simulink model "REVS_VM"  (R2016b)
settings: Solver=ode3  StartTime=REVS.sim_start_time_secs  StopTime=Inf  FixedStep=REVS.sim_step_time_secs  MaxStep=REVS.sim_step_time_secs  EnableMultiTasking=on
StopFcn:
  | postproc_datalog;
  | postproc_audit;
  | postproc_result;
model workspace (MATLAB code in the model file):
  other statements: REVS_setup_variants
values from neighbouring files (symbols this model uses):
  accessory = class_accessory_data    [class_test_data.m]
  battery = class_battery_data    [class_accessory_data.m]    (also in class_REVS_electric.m = class_REVS_battery)
  brake = struct(	'max_torque_Nm',[], 						'proportion_norm',1.0, 						'inertia_kgm2',0.0)    [class_REVS_drive_axle.m]
  engine = class_engine_data    [class_test_data.m]
  final_drive = struct(	'gear_ratio',[], 								'efficiency_norm',[], 								'inertia_kgm2',[] )    [class_REVS_drive_axle.m]
  gear = class_REVS_gearbox    [class_REVS_AT_transmission.m]
  tire = struct(	'radius_m',[], 						'rolling_resistance_coefficient',0, 						'vehicle_weight_norm',1.0,  						'wheel_slip_torque_Nm',[],  						'inertia_kgm2',0.0)    [class_REVS_drive_axle.m]
  torque_converter = class_REVS_torque_converter    [class_REVS_AT_transmission.m]
  transmission = class_transmission_data    [class_test_data.m]
  vehicle = class_vehicle_data    [class_test_data.m]
undefined symbols (not defined in the file or in its folder): alternator, ambient, controls, convert, DelayTimeSecs, drive_cycle, driver, electric, gear_strategy, InitialCondition, InitialValue, LoadSource, LookupStructure, MultiplyPosInputs, Normalize, NumPhases, REVS, SpeedSource, starter, tableshift, UpperSaturationLimit, Value, VerboseLevel, VerboseSignal
libraries: simulink x153
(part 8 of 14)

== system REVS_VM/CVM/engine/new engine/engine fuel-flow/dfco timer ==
  bool : Inport
  Constant : Constant  Value=Normalize
  Data Type Conversion2 : DataTypeConversion  OutDataTypeStr=double
  Integrator1 : Integrator  ExternalReset=falling  LimitOutput=on  UpperSaturationLimit=UpperSaturationLimit  LowerSaturationLimit=0
  Switch : Switch  Criteria=u2 > Threshold
  normalize : Gain  Gain=1/UpperSaturationLimit
  out : Outport
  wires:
  Switch/1 -> out/1
  normalize/1 -> Switch/1
  Integrator1/1 -> Switch/3, normalize/1
  Constant/1 -> Switch/2
  bool/1 -> Data Type Conversion2/1
  Data Type Conversion2/1 -> Integrator1/1, Integrator1/2

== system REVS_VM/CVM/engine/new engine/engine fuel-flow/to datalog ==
  Var : Inport
  Constant : Constant  Value=VerboseSignal
  Constant1 : Constant  Value=VerboseLevel
  Relational Operator : RelationalOperator  OutDataTypeStr=boolean  ZeroCross=off
  Subsystem : Subsystem
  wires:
  Constant1/1 -> Relational Operator/2
  Constant/1 -> Relational Operator/1
  Relational Operator/1 -> Subsystem/Enable
  Var/1 -> Subsystem/1(In1)

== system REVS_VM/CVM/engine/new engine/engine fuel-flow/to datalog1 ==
  Var : Inport
  Constant : Constant  Value=VerboseSignal
  Constant1 : Constant  Value=VerboseLevel
  Relational Operator : RelationalOperator  OutDataTypeStr=boolean  ZeroCross=off
  Subsystem : Subsystem
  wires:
  Constant1/1 -> Relational Operator/2
  Constant/1 -> Relational Operator/1
  Relational Operator/1 -> Subsystem/Enable
  Var/1 -> Subsystem/1(In1)

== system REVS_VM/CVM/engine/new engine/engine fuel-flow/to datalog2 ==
  Var : Inport
  Constant : Constant  Value=VerboseSignal
  Constant1 : Constant  Value=VerboseLevel
  Relational Operator : RelationalOperator  OutDataTypeStr=boolean  ZeroCross=off
  Subsystem : Subsystem
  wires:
  Constant1/1 -> Relational Operator/2
  Constant/1 -> Relational Operator/1
  Relational Operator/1 -> Subsystem/Enable
  Var/1 -> Subsystem/1(In1)

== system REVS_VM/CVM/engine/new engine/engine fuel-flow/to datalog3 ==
  Var : Inport
  Constant : Constant  Value=VerboseSignal
  Constant1 : Constant  Value=VerboseLevel
  Relational Operator : RelationalOperator  OutDataTypeStr=boolean  ZeroCross=off
  Subsystem : Subsystem
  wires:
  Constant1/1 -> Relational Operator/2
  Constant/1 -> Relational Operator/1
  Relational Operator/1 -> Subsystem/Enable
  Var/1 -> Subsystem/1(In1)

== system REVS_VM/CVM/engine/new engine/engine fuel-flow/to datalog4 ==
  Var : Inport
  Constant : Constant  Value=VerboseSignal
  Constant1 : Constant  Value=VerboseLevel
  Relational Operator : RelationalOperator  OutDataTypeStr=boolean  ZeroCross=off
  Subsystem : Subsystem
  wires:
  Constant1/1 -> Relational Operator/2
  Constant/1 -> Relational Operator/1
  Relational Operator/1 -> Subsystem/Enable
  Var/1 -> Subsystem/1(In1)

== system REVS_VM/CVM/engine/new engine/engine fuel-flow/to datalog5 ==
  Var : Inport
  Constant : Constant  Value=VerboseSignal
  Constant1 : Constant  Value=VerboseLevel
  Relational Operator : RelationalOperator  OutDataTypeStr=boolean  ZeroCross=off
  Subsystem : Subsystem
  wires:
  Constant1/1 -> Relational Operator/2
  Constant/1 -> Relational Operator/1
  Relational Operator/1 -> Subsystem/Enable
  Var/1 -> Subsystem/1(In1)

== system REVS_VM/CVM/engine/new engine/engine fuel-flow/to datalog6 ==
  Var : Inport
  Constant : Constant  Value=VerboseSignal
  Constant1 : Constant  Value=VerboseLevel
  Relational Operator : RelationalOperator  OutDataTypeStr=boolean  ZeroCross=off
  Subsystem : Subsystem
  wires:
  Constant1/1 -> Relational Operator/2
  Constant/1 -> Relational Operator/1
  Relational Operator/1 -> Subsystem/Enable
  Var/1 -> Subsystem/1(In1)

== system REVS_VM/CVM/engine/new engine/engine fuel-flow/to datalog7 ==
  Var : Inport
  Constant : Constant  Value=VerboseSignal
  Constant1 : Constant  Value=VerboseLevel
  Relational Operator : RelationalOperator  OutDataTypeStr=boolean  ZeroCross=off
  Subsystem : Subsystem
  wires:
  Constant1/1 -> Relational Operator/2
  Constant/1 -> Relational Operator/1
  Relational Operator/1 -> Subsystem/Enable
  Var/1 -> Subsystem/1(In1)

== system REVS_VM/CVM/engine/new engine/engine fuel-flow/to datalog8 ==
  Var : Inport
  Constant : Constant  Value=VerboseSignal
  Constant1 : Constant  Value=VerboseLevel
  Relational Operator : RelationalOperator  OutDataTypeStr=boolean  ZeroCross=off
  Subsystem : Subsystem
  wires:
  Constant1/1 -> Relational Operator/2
  Constant/1 -> Relational Operator/1
  Relational Operator/1 -> Subsystem/Enable
  Var/1 -> Subsystem/1(In1)

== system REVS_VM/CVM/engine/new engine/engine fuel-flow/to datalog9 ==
  Var : Inport
  Constant : Constant  Value=VerboseSignal
  Constant1 : Constant  Value=VerboseLevel
  Relational Operator : RelationalOperator  OutDataTypeStr=boolean  ZeroCross=off
  Subsystem : Subsystem
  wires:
  Constant1/1 -> Relational Operator/2
  Constant/1 -> Relational Operator/1
  Relational Operator/1 -> Subsystem/Enable
  Var/1 -> Subsystem/1(In1)

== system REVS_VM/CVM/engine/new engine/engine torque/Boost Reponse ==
  target_trq_Nm : Inport
  max_trq_Nm : Inport  Port=2
  nat_asp_trq_Nm : Inport  Port=3
  min_trq_Nm : Inport  Port=4
  Constant : Constant  Value=engine.boost_time_constant_secs
  Constant1 : Constant  Value=engine.boost_falling_time_constant_secs
  Dynamic Limit Integrator : Subsystem
  MinMax3 : MinMax  Function=max  Inputs=2  ZeroCross=off
  MinMax4 : MinMax  Inputs=2  ZeroCross=off
  Product : Product  Inputs=*/
  Sum : Sum  Inputs=|+-
  Sum1 : Sum  Inputs=|+-
  Switch : Switch  Criteria=u2 > Threshold
  trq_limit_Nm : Outport
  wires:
  min_trq_Nm/1 -> Sum1/2
  nat_asp_trq_Nm/1 -> Sum1/1
  Constant1/1 -> Switch/3
  Constant/1 -> Switch/1
  Switch/1 -> Product/2
  target_trq_Nm/1 -> MinMax3/1
  max_trq_Nm/1 -> Dynamic Limit Integrator/1(upper), MinMax4/1
  Sum1/1 -> MinMax3/2, Dynamic Limit Integrator/4(Xo), Dynamic Limit Integrator/5(lower)
  Product/1 -> Dynamic Limit Integrator/2(In)
  MinMax4/1 -> Sum/1
  Sum/1 -> Switch/2, Product/1
  MinMax3/1 -> MinMax4/2
  Dynamic Limit Integrator/1(Out) -> trq_limit_Nm/1, Sum/2

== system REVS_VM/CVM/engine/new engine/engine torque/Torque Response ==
  target_pow_W : Inport
  Constant : Constant  Value=1/engine.power_time_constant_secs
  Integrator : Integrator
  Product : Product
  Sum : Sum  Inputs=|+-
  act_pow_W : Outport
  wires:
  Product/1 -> Integrator/1
  Constant/1 -> Product/1
  Integrator/1 -> Sum/2, act_pow_W/1
  Sum/1 -> Product/2
  target_pow_W/1 -> Sum/1

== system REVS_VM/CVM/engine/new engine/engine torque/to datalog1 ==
  Var : Inport
  Constant : Constant  Value=VerboseSignal
  Constant1 : Constant  Value=VerboseLevel
  Relational Operator : RelationalOperator  OutDataTypeStr=boolean  ZeroCross=off
  Subsystem : Subsystem
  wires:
  Constant1/1 -> Relational Operator/2
  Constant/1 -> Relational Operator/1
  Relational Operator/1 -> Subsystem/Enable
  Var/1 -> Subsystem/1(In1)

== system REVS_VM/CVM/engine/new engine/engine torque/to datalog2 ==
  Var : Inport
  Constant : Constant  Value=VerboseSignal
  Constant1 : Constant  Value=VerboseLevel
  Relational Operator : RelationalOperator  OutDataTypeStr=boolean  ZeroCross=off
  Subsystem : Subsystem
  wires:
  Constant1/1 -> Relational Operator/2
  Constant/1 -> Relational Operator/1
  Relational Operator/1 -> Subsystem/Enable
  Var/1 -> Subsystem/1(In1)

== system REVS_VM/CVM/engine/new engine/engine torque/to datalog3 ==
  Var : Inport
  Constant : Constant  Value=VerboseSignal
  Constant1 : Constant  Value=VerboseLevel
  Relational Operator : RelationalOperator  OutDataTypeStr=boolean  ZeroCross=off
  Subsystem : Subsystem
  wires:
  Constant1/1 -> Relational Operator/2
  Constant/1 -> Relational Operator/1
  Relational Operator/1 -> Subsystem/Enable
  Var/1 -> Subsystem/1(In1)

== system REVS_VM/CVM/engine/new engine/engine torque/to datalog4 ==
  Var : Inport
  Constant : Constant  Value=VerboseSignal
  Constant1 : Constant  Value=VerboseLevel
  Relational Operator : RelationalOperator  OutDataTypeStr=boolean  ZeroCross=off
  Subsystem : Subsystem
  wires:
  Constant1/1 -> Relational Operator/2
  Constant/1 -> Relational Operator/1
  Relational Operator/1 -> Subsystem/Enable
  Var/1 -> Subsystem/1(In1)

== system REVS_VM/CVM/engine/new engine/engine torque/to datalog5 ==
  Var : Inport
  Constant : Constant  Value=VerboseSignal
  Constant1 : Constant  Value=VerboseLevel
  Relational Operator : RelationalOperator  OutDataTypeStr=boolean  ZeroCross=off
  Subsystem : Subsystem
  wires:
  Constant1/1 -> Relational Operator/2
  Constant/1 -> Relational Operator/1
  Relational Operator/1 -> Subsystem/Enable
  Var/1 -> Subsystem/1(In1)

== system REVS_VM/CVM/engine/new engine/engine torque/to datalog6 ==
  Var : Inport
  Constant : Constant  Value=VerboseSignal
  Constant1 : Constant  Value=VerboseLevel
  Relational Operator : RelationalOperator  OutDataTypeStr=boolean  ZeroCross=off
  Subsystem : Subsystem
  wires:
  Constant1/1 -> Relational Operator/2
  Constant/1 -> Relational Operator/1
  Relational Operator/1 -> Subsystem/Enable
  Var/1 -> Subsystem/1(In1)

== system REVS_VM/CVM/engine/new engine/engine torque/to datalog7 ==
  Var : Inport
  Constant : Constant  Value=VerboseSignal
  Constant1 : Constant  Value=VerboseLevel
  Relational Operator : RelationalOperator  OutDataTypeStr=boolean  ZeroCross=off
  Subsystem : Subsystem
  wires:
  Constant1/1 -> Relational Operator/2
  Constant/1 -> Relational Operator/1
  Relational Operator/1 -> Subsystem/Enable
  Var/1 -> Subsystem/1(In1)

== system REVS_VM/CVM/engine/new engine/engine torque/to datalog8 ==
  Var : Inport
  Constant : Constant  Value=VerboseSignal
  Constant1 : Constant  Value=VerboseLevel
  Relational Operator : RelationalOperator  OutDataTypeStr=boolean  ZeroCross=off
  Subsystem : Subsystem
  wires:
  Constant1/1 -> Relational Operator/2
  Constant/1 -> Relational Operator/1
  Relational Operator/1 -> Subsystem/Enable
  Var/1 -> Subsystem/1(In1)

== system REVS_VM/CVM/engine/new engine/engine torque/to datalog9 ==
  Var : Inport
  Constant : Constant  Value=VerboseSignal
  Constant1 : Constant  Value=VerboseLevel
  Relational Operator : RelationalOperator  OutDataTypeStr=boolean  ZeroCross=off
  Subsystem : Subsystem
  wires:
  Constant1/1 -> Relational Operator/2
  Constant/1 -> Relational Operator/1
  Relational Operator/1 -> Subsystem/Enable
  Var/1 -> Subsystem/1(In1)

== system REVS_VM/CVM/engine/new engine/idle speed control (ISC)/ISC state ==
  eng_on : Inport
  eng_spd_radps : Inport  Port=2
  Compare To Constant : simulink/Logic and Bit Operations/Compare To Constant  relop=>  const=0.5  OutDataTypeStr=boolean
  Compare To Zero : simulink/Logic and Bit Operations/Compare To Zero  relop===  OutDataTypeStr=boolean
  Data Type Conversion2 : DataTypeConversion
  Latch : Subsystem
  Logical Operator : Logic  AllPortsSameDT=off  OutDataTypeStr=boolean
  Logical Operator1 : Logic  Operator=OR  AllPortsSameDT=off  OutDataTypeStr=boolean
  Relational Operator : RelationalOperator  Operator=>  OutDataTypeStr=boolean
  Relational Operator1 : RelationalOperator  Operator=<  OutDataTypeStr=boolean
  activation_speed_radps : Constant  Value=engine.idle_control_activation_speed_radps
  boolean integrator : Subsystem
  deactivation_speed_radps : Constant  Value=engine.idle_control_deactivation_speed_radps
  state : Outport
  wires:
  Relational Operator/1 -> Logical Operator/2
  boolean integrator/1(out) -> Compare To Constant/1
  eng_spd_radps/1 -> Relational Operator1/1, Relational Operator/1
  activation_speed_radps/1 -> Relational Operator/2
  Logical Operator1/1 -> Latch/2(Off)
  Compare To Constant/1 -> Latch/1(On)
  deactivation_speed_radps/1 -> Relational Operator1/2
  Latch/1(State) -> Data Type Conversion2/1
  Data Type Conversion2/1 -> state/1
  Logical Operator/1 -> boolean integrator/1(bool)
  eng_on/1 -> Compare To Zero/1, Logical Operator/1
  Relational Operator1/1 -> Logical Operator1/1
  Compare To Zero/1 -> Logical Operator1/2

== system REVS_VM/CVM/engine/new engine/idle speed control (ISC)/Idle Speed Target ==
  system_bus : Inport
  eng_spd_radps : Inport  Port=2
  eng_des_spd_radps : Inport  Port=3
  ISC_state : Inport  Port=4
  Data Type Conversion : DataTypeConversion
  MinMax : MinMax  Function=max  Inputs=2
  Product1 : Product
  Rate Limiter : RateLimiter  RisingSlewLimit=1/engine.idle_control_ramp_time_secs  FallingSlewLimit=-1/engine.idle_control_ramp_time_secs  SampleTimeMode=inherited
  Relational Operator : RelationalOperator  OutDataTypeStr=boolean
  Sum1 : Sum
  Sum3 : Sum
  idle ramp : Product
  running timer : Integrator  ExternalReset=falling
  soft landing offset radps : Constant  Value=engine.idle_control_ramp_radps
  startup flare : Lookup_n-D  NumberOfTableDimensions=1  BreakpointsForDimension1=[0 0.5 1.25 2.25 3.0 3.5]  IndexSearchMethod=Linear search  Table="[0.5 1.1 1.2 1.2  1.1 1.0]"  InterpMethod=Cubic spline  ExtrapMethod=Clip  RndMeth=Simplest
  target idle speed : Subsystem
  target_idle_spd_radps : Outport
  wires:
  system_bus/1 -> target idle speed/1(bus)
  eng_spd_radps/1 -> Relational Operator/1
  ISC_state/1 -> running timer/2, running timer/1
  startup flare/1 -> Product1/1
  eng_des_spd_radps/1 -> MinMax/1
  target idle speed/1(out) -> Product1/2
  MinMax/1 -> Sum1/2, Sum3/2
  Product1/1 -> MinMax/2
  running timer/1 -> startup flare/1
  Relational Operator/1 -> Data Type Conversion/1
  soft landing offset radps/1 -> idle ramp/1, Sum3/1
  Rate Limiter/1 -> idle ramp/2
  Sum3/1 -> Relational Operator/2
  idle ramp/1 -> Sum1/1
  Data Type Conversion/1 -> Rate Limiter/1
  Sum1/1 -> target_idle_spd_radps/1

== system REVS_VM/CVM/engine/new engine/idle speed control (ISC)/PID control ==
  ISC_state : Inport
  error : Inport  Port=2
  Derivative : Derivative
  Integrator : Integrator  ExternalReset=level  LimitOutput=on  UpperSaturationLimit=Inf  LowerSaturationLimit=0
  Kd : Gain  Gain=engine.idle_control_Kd
  Ki : Gain  Gain=engine.idle_control_Ki
  Kp : Gain  Gain=engine.idle_control_Kp
  Logical Operator : Logic  Operator=NOT  AllPortsSameDT=off  OutDataTypeStr=boolean
  Product1 : Product
  Product2 : Product
  Subtract : Sum  Inputs=+++
  sat >= 0 : Saturate  UpperLimit=Inf  LowerLimit=0  ZeroCross=off
  to datalog2 : Subsystem
  to datalog3 : Subsystem
  PID_trq_Nm : Outport
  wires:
  Subtract/1 -> PID_trq_Nm/1
  Product1/1 -> to datalog3/1(Var)
  ISC_state/1 -> Logical Operator/1, Product2/1, Product1/1
  Product2/1 -> to datalog2/1(Var)
  Logical Operator/1 -> Integrator/2
  Kd/1 -> sat >= 0/1
  Ki/1 -> Integrator/1
  Derivative/1 -> Subtract/3
  Integrator/1 -> Product2/2, Subtract/2
  error/1 -> Kd/1, Ki/1, Kp/1
  sat >= 0/1 -> Derivative/1
  Kp/1 -> Product1/2, Subtract/1

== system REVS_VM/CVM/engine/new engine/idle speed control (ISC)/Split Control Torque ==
  ISC_state : Inport
  ISC_trq : Inport  Port=2
  Add1 : Sum  Inputs=-+|
  Add2 : Sum  Inputs=|++
  Add3 : Sum  Inputs=|+-
  Constant : Constant  Value=engine.idle_control_torque_reserve_Nm
  Fcn : Fcn  Expr="u * ( 1  +  10*( u <0 ) )/engine.power_time_constant_secs"
  Integrator1 : Integrator
  MinMax : MinMax  Function=max  Inputs=2
  Product1 : Product
  Product3 : Product
  neg : Gain  Gain=-1.1
  pos : Saturate  UpperLimit=inf  LowerLimit=0  ZeroCross=off
  pos1 : Saturate  UpperLimit=inf  LowerLimit=0  ZeroCross=off
  to datalog1 : Subsystem
  to datalog9 : Subsystem
  ISC_slow_trq : Outport
  ISC_fast_trq : Outport  Port=2
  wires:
  Product1/1 -> pos1/1
  Add2/1 -> Product3/2
  ISC_state/1 -> Product3/1, Product1/1
  neg/1 -> MinMax/2
  Add1/1 -> MinMax/1
  Add3/1 -> Fcn/1
  Fcn/1 -> Integrator1/1
  pos/1 -> ISC_slow_trq/1, Add3/1
  Integrator1/1 -> to datalog9/1(Var), Add3/2, Add1/1
  Product3/1 -> pos/1
  pos1/1 -> to datalog1/1(Var), Add1/2
  Constant/1 -> Add2/2, neg/1
  MinMax/1 -> ISC_fast_trq/1
  ISC_trq/1 -> Product1/2, Add2/1

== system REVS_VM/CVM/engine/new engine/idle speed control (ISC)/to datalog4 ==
  Var : Inport
  Constant : Constant  Value=VerboseSignal
  Constant1 : Constant  Value=VerboseLevel
  Relational Operator : RelationalOperator  OutDataTypeStr=boolean  ZeroCross=off
  Subsystem : Subsystem
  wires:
  Constant1/1 -> Relational Operator/2
  Constant/1 -> Relational Operator/1
  Relational Operator/1 -> Subsystem/Enable
  Var/1 -> Subsystem/1(In1)

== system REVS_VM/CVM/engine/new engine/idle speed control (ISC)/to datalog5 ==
  Var : Inport
  Constant : Constant  Value=VerboseSignal
  Constant1 : Constant  Value=VerboseLevel
  Relational Operator : RelationalOperator  OutDataTypeStr=boolean  ZeroCross=off
  Subsystem : Subsystem
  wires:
  Constant1/1 -> Relational Operator/2
  Constant/1 -> Relational Operator/1
  Relational Operator/1 -> Subsystem/Enable
  Var/1 -> Subsystem/1(In1)

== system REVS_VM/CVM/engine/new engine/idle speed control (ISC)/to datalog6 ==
  Var : Inport
  Constant : Constant  Value=VerboseSignal
  Constant1 : Constant  Value=VerboseLevel
  Relational Operator : RelationalOperator  OutDataTypeStr=boolean  ZeroCross=off
  Subsystem : Subsystem
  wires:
  Constant1/1 -> Relational Operator/2
  Constant/1 -> Relational Operator/1
  Relational Operator/1 -> Subsystem/Enable
  Var/1 -> Subsystem/1(In1)

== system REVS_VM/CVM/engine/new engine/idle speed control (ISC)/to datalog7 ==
  Var : Inport
  Constant : Constant  Value=VerboseSignal
  Constant1 : Constant  Value=VerboseLevel
  Relational Operator : RelationalOperator  OutDataTypeStr=boolean  ZeroCross=off
  Subsystem : Subsystem
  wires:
  Constant1/1 -> Relational Operator/2
  Constant/1 -> Relational Operator/1
  Relational Operator/1 -> Subsystem/Enable
  Var/1 -> Subsystem/1(In1)

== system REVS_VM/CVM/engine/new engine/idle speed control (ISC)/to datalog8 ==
  Var : Inport
  Constant : Constant  Value=VerboseSignal
  Constant1 : Constant  Value=VerboseLevel
  Relational Operator : RelationalOperator  OutDataTypeStr=boolean  ZeroCross=off
  Subsystem : Subsystem
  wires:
  Constant1/1 -> Relational Operator/2
  Constant/1 -> Relational Operator/1
  Relational Operator/1 -> Subsystem/Enable
  Var/1 -> Subsystem/1(In1)

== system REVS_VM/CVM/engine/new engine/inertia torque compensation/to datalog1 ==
  Var : Inport
  Constant : Constant  Value=VerboseSignal
  Constant1 : Constant  Value=VerboseLevel
  Relational Operator : RelationalOperator  OutDataTypeStr=boolean  ZeroCross=off
  Subsystem : Subsystem
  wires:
  Constant1/1 -> Relational Operator/2
  Constant/1 -> Relational Operator/1
  Relational Operator/1 -> Subsystem/Enable
  Var/1 -> Subsystem/1(In1)

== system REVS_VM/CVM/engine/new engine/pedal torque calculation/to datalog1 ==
  Var : Inport
  Constant : Constant  Value=VerboseSignal
  Constant1 : Constant  Value=VerboseLevel
  Relational Operator : RelationalOperator  OutDataTypeStr=boolean  ZeroCross=off
  Subsystem : Subsystem
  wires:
  Constant1/1 -> Relational Operator/2
  Constant/1 -> Relational Operator/1
  Relational Operator/1 -> Subsystem/Enable
  Var/1 -> Subsystem/1(In1)

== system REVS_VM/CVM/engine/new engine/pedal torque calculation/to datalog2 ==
  Var : Inport
  Constant : Constant  Value=VerboseSignal
  Constant1 : Constant  Value=VerboseLevel
  Relational Operator : RelationalOperator  OutDataTypeStr=boolean  ZeroCross=off
  Subsystem : Subsystem
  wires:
  Constant1/1 -> Relational Operator/2
  Constant/1 -> Relational Operator/1
  Relational Operator/1 -> Subsystem/Enable
  Var/1 -> Subsystem/1(In1)

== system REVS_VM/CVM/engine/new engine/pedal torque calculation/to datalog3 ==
  Var : Inport
  Constant : Constant  Value=VerboseSignal
  Constant1 : Constant  Value=VerboseLevel
  Relational Operator : RelationalOperator  OutDataTypeStr=boolean  ZeroCross=off
  Subsystem : Subsystem
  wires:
  Constant1/1 -> Relational Operator/2
  Constant/1 -> Relational Operator/1
  Relational Operator/1 -> Subsystem/Enable
  Var/1 -> Subsystem/1(In1)

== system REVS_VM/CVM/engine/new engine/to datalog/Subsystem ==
  In1 : Inport
  Enable : EnablePort
  To Workspace : ToWorkspace  VariableName=datalog__engine__fuel_rate_gps  SampleTime=-1
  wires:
  In1/1 -> To Workspace/1

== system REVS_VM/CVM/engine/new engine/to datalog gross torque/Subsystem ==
  In1 : Inport
  Enable : EnablePort
  To Workspace : ToWorkspace  VariableName=datalog__engine__crankshaft_gross_torque_Nm  SampleTime=-1
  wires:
  In1/1 -> To Workspace/1

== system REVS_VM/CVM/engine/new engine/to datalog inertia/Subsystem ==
  In1 : Inport
  Enable : EnablePort
  To Workspace : ToWorkspace  VariableName=datalog__engine__crankshaft_gross_inertia_kgm2  SampleTime=-1
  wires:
  In1/1 -> To Workspace/1

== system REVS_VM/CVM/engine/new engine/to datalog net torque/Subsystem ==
  In1 : Inport
  Enable : EnablePort
  To Workspace : ToWorkspace  VariableName=datalog__engine__crankshaft_torque_Nm  SampleTime=-1
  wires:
  In1/1 -> To Workspace/1

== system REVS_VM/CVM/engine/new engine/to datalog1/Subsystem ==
  In1 : Inport
  Enable : EnablePort
  To Workspace : ToWorkspace  VariableName=datalog__engine__fuel_consumed_g  SampleTime=-1
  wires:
  In1/1 -> To Workspace/1

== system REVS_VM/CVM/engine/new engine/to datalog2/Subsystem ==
  In1 : Inport
  Enable : EnablePort
  To Workspace : ToWorkspace  VariableName=datalog__engine__deac_active_norm  SampleTime=-1
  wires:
  In1/1 -> To Workspace/1

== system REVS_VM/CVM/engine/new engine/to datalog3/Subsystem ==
  In1 : Inport
  Enable : EnablePort
  To Workspace : ToWorkspace  VariableName=datalog__engine__DFCO_active_bool  SampleTime=-1
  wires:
  In1/1 -> To Workspace/1

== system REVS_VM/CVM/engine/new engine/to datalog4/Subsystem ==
  In1 : Inport
  Enable : EnablePort
  To Workspace : ToWorkspace  VariableName=datalog__engine__crankshaft_speed_radps  SampleTime=-1
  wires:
  In1/1 -> To Workspace/1

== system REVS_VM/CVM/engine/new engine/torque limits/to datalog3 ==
  Var : Inport
  Constant : Constant  Value=VerboseSignal
  Constant1 : Constant  Value=VerboseLevel
  Relational Operator : RelationalOperator  OutDataTypeStr=boolean  ZeroCross=off
  Subsystem : Subsystem
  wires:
  Constant1/1 -> Relational Operator/2
  Constant/1 -> Relational Operator/1
  Relational Operator/1 -> Subsystem/Enable
  Var/1 -> Subsystem/1(In1)

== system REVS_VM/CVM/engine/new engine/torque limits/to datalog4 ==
  Var : Inport
  Constant : Constant  Value=VerboseSignal
  Constant1 : Constant  Value=VerboseLevel
  Relational Operator : RelationalOperator  OutDataTypeStr=boolean  ZeroCross=off
  Subsystem : Subsystem
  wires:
  Constant1/1 -> Relational Operator/2
  Constant/1 -> Relational Operator/1
  Relational Operator/1 -> Subsystem/Enable
  Var/1 -> Subsystem/1(In1)

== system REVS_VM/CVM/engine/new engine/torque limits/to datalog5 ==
  Var : Inport
  Constant : Constant  Value=VerboseSignal
  Constant1 : Constant  Value=VerboseLevel
  Relational Operator : RelationalOperator  OutDataTypeStr=boolean  ZeroCross=off
  Subsystem : Subsystem
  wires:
  Constant1/1 -> Relational Operator/2
  Constant/1 -> Relational Operator/1
  Relational Operator/1 -> Subsystem/Enable
  Var/1 -> Subsystem/1(In1)

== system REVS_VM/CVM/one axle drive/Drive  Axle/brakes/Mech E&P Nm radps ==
  " trq_Nm" : Inport
  spd_radps : Inport  Port=2
  iner_kgm2 : Inport  Port=3
  Compare To Constant : simulink/Logic and Bit Operations/Compare To Constant  relop=>=  const=1  OutDataTypeStr=boolean
  Constant : Constant  Value=VerboseSignal
  Subsystem : Subsystem
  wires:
  " trq_Nm"/1 -> Subsystem/1(" trq_Nm")
  spd_radps/1 -> Subsystem/2(spd_radps)
  iner_kgm2/1 -> Subsystem/3(iner_kgm2)
  Compare To Constant/1 -> Subsystem/Enable
  Constant/1 -> Compare To Constant/1

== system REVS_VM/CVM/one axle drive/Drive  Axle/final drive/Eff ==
  Efficiency : Inport
  Input : Inport  Port=2
  Math Function : Math  Operator=reciprocal
  Product1 : Product
  Switch : Switch  ZeroCross=off
  Output : Outport
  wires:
  Math Function/1 -> Switch/3
  Product1/1 -> Output/1
  Input/1 -> Product1/2, Switch/2
  Efficiency/1 -> Switch/1, Math Function/1
  Switch/1 -> Product1/1

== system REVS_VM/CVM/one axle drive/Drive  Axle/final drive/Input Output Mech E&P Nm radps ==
  trq_in_Nm : Inport
  spd_in_radps : Inport  Port=2
  iner_in_kgm2 : Inport  Port=3
  trq_out_Nm : Inport  Port=4
  spd_out_radps : Inport  Port=5
  iner_out_kgm2 : Inport  Port=6
  Compare To Constant : simulink/Logic and Bit Operations/Compare To Constant  relop=>=  const=1  OutDataTypeStr=boolean
  Constant : Constant  Value=VerboseSignal
  Subsystem : Subsystem
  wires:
  trq_in_Nm/1 -> Subsystem/1(trq_in_Nm)
  spd_in_radps/1 -> Subsystem/2(spd_in_radps)
  iner_in_kgm2/1 -> Subsystem/3(iner_in_kgm2)
  trq_out_Nm/1 -> Subsystem/4(trq_out_Nm)
  spd_out_radps/1 -> Subsystem/5(spd_out_radps)
  iner_out_kgm2/1 -> Subsystem/6(iner_out_kgm2)
  Compare To Constant/1 -> Subsystem/Enable
  Constant/1 -> Compare To Constant/1

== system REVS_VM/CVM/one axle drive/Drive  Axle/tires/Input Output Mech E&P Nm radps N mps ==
  trq_in_Nm : Inport
  spd_in_radps : Inport  Port=2
  iner_in_kgm2 : Inport  Port=3
  frc_out_N : Inport  Port=4
  spd_out_mps : Inport  Port=5
  mass_out_kg : Inport  Port=6
  Compare To Constant : simulink/Logic and Bit Operations/Compare To Constant  relop=>=  const=1  OutDataTypeStr=boolean
  Constant : Constant  Value=VerboseSignal
  Subsystem : Subsystem
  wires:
  Constant/1 -> Compare To Constant/1
  Compare To Constant/1 -> Subsystem/Enable
  mass_out_kg/1 -> Subsystem/6(mass_out_kg)
  spd_out_mps/1 -> Subsystem/5(spd_out_mps)
  frc_out_N/1 -> Subsystem/4(frc_out_N)
  iner_in_kgm2/1 -> Subsystem/3(iner_in_kgm2)
  spd_in_radps/1 -> Subsystem/2(spd_in_radps)
  trq_in_Nm/1 -> Subsystem/1(trq_in_Nm)

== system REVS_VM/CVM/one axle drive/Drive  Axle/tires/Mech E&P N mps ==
  force_N : Inport
  spd_mps : Inport  Port=2
  Compare To Constant : simulink/Logic and Bit Operations/Compare To Constant  relop=>=  const=1  OutDataTypeStr=boolean
  Constant : Constant  Value=VerboseSignal
  Subsystem : Subsystem
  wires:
  Constant/1 -> Compare To Constant/1
  Compare To Constant/1 -> Subsystem/Enable
  spd_mps/1 -> Subsystem/2(spd_mps)
  force_N/1 -> Subsystem/1(force_N)

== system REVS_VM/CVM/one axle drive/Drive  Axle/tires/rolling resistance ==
  system_bus : Inport
  veh_spd_mps : Inport  Port=2
  Crr : Inport  Port=3
  % grade to norm : Gain  Gain=0.01
  Bus Selector : BusSelector  OutputSignals=ambient.drive_cycle_grade_pct
  Gravitational Acceleration (m/sec^2)1 : Constant  Value=ambient.gravity_mps2
  Rolling Resistance Force (N) : Product  Inputs=5
  Sign : Lookup_n-D  NumberOfTableDimensions=1  BreakpointsForDimension1=[-eps 0 eps]  BeginIndexSearchUsingPreviousIndexResult=on  Table=[-1 1 1]  ExtrapMethod=Clip  UseLastTableValue=on  RndMeth=Simplest
  Static Vehicle Mass (kg) : Constant  Value=vehicle.mass_static_kg
  Sum : Sum  Inputs=|++
  Trigonometric Function2 : Trigonometry  Operator=atan
  Trigonometric Function3 : Trigonometry  Operator=cos
  dynamic lookup : Subsystem
  " roll_res_force_N" : Outport
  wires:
  Static Vehicle Mass (kg)/1 -> Sum/2
  dynamic lookup/1(out) -> Sum/1
  Sum/1 -> Rolling Resistance Force (N)/3
  system_bus/1 -> dynamic lookup/1(bus), Bus Selector/1
  Bus Selector/1 -> % grade to norm/1  "<drive_cycle_grade_pct>"
  Sign/1 -> Rolling Resistance Force (N)/4
  Crr/1 -> Rolling Resistance Force (N)/5
  Rolling Resistance Force (N)/1 -> " roll_res_force_N"/1
  Trigonometric Function3/1 -> Rolling Resistance Force (N)/1
  % grade to norm/1 -> Trigonometric Function2/1
  Gravitational Acceleration (m/sec^2)1/1 -> Rolling Resistance Force (N)/2
  Trigonometric Function2/1 -> Trigonometric Function3/1
  veh_spd_mps/1 -> Sign/1

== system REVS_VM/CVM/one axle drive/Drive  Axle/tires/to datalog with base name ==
  Var : Inport
  Constant : Constant  Value=VerboseSignal
  Constant1 : Constant  Value=VerboseLevel
  Relational Operator : RelationalOperator  OutDataTypeStr=boolean  ZeroCross=off
  Subsystem : Subsystem
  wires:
  Constant1/1 -> Relational Operator/2
  Relational Operator/1 -> Subsystem/Enable
  Constant/1 -> Relational Operator/1
  Var/1 -> Subsystem/1(Var)

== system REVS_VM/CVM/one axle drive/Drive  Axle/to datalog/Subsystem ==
  In1 : Inport
  Enable : EnablePort
  To Workspace : ToWorkspace  VariableName=datalog__final_drive__output_torque_Nm  SampleTime=-1
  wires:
  In1/1 -> To Workspace/1

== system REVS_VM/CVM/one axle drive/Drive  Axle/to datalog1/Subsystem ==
  In1 : Inport
  Enable : EnablePort
  To Workspace : ToWorkspace  VariableName=datalog__final_drive__output_inertia_kgm2  SampleTime=-1
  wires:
  In1/1 -> To Workspace/1

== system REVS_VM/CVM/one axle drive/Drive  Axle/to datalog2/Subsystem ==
  In1 : Inport
  Enable : EnablePort
  To Workspace : ToWorkspace  VariableName=datalog__final_drive__output_speed_radps  SampleTime=-1
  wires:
  In1/1 -> To Workspace/1

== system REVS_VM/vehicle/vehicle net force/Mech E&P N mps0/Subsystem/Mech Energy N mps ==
  force_N : Inport
  spd_mps : Inport  Port=2
  Gain : Gain  Gain=-1
  Integrator : Integrator  ZeroCross=off
  Integrator1 : Integrator  ZeroCross=off
  Integrator2 : Integrator  ZeroCross=off
  Mux : Mux  Inputs=2
  Neg : Fcn  Expr=u(1)*(u(1) <= 0)
  Pos : Fcn  Expr=u(1)*(u(1) >= 0)
  calc_Power_kW : Fcn  Expr=u(1)*u(2)/1000
  "total_kJ " : Outport
  "pos_kJ " : Outport  Port=2
  neg_kJ : Outport  Port=3
  pwr_kW : Outport  Port=4
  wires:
  calc_Power_kW/1 -> Pos/1, Neg/1, pwr_kW/1, Integrator/1
  Gain/1 -> neg_kJ/1
  Integrator1/1 -> "pos_kJ "/1
  Integrator2/1 -> Gain/1
  Neg/1 -> Integrator2/1
  Pos/1 -> Integrator1/1
  Integrator/1 -> "total_kJ "/1
  Mux/1 -> calc_Power_kW/1
  force_N/1 -> Mux/1
  spd_mps/1 -> Mux/2

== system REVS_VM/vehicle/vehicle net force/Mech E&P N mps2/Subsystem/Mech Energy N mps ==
  force_N : Inport
  spd_mps : Inport  Port=2
  Gain : Gain  Gain=-1
  Integrator : Integrator  ZeroCross=off
  Integrator1 : Integrator  ZeroCross=off
  Integrator2 : Integrator  ZeroCross=off
  Mux : Mux  Inputs=2
  Neg : Fcn  Expr=u(1)*(u(1) <= 0)
  Pos : Fcn  Expr=u(1)*(u(1) >= 0)
  calc_Power_kW : Fcn  Expr=u(1)*u(2)/1000
  "total_kJ " : Outport
  "pos_kJ " : Outport  Port=2
  neg_kJ : Outport  Port=3
  pwr_kW : Outport  Port=4
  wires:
  calc_Power_kW/1 -> Pos/1, Neg/1, pwr_kW/1, Integrator/1
  Gain/1 -> neg_kJ/1
  Integrator1/1 -> "pos_kJ "/1
  Integrator2/1 -> Gain/1
  Neg/1 -> Integrator2/1
  Pos/1 -> Integrator1/1
  Integrator/1 -> "total_kJ "/1
  Mux/1 -> calc_Power_kW/1
  force_N/1 -> Mux/1
  spd_mps/1 -> Mux/2

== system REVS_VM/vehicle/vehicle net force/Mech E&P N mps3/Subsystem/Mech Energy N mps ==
  force_N : Inport
  spd_mps : Inport  Port=2
  Gain : Gain  Gain=-1
  Integrator : Integrator  ZeroCross=off
  Integrator1 : Integrator  ZeroCross=off
  Integrator2 : Integrator  ZeroCross=off
  Mux : Mux  Inputs=2
  Neg : Fcn  Expr=u(1)*(u(1) <= 0)
  Pos : Fcn  Expr=u(1)*(u(1) >= 0)
  calc_Power_kW : Fcn  Expr=u(1)*u(2)/1000
  "total_kJ " : Outport
  "pos_kJ " : Outport  Port=2
  neg_kJ : Outport  Port=3
  pwr_kW : Outport  Port=4
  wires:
  calc_Power_kW/1 -> Pos/1, Neg/1, pwr_kW/1, Integrator/1
  Gain/1 -> neg_kJ/1
  Integrator1/1 -> "pos_kJ "/1
  Integrator2/1 -> Gain/1
  Neg/1 -> Integrator2/1
  Pos/1 -> Integrator1/1
  Integrator/1 -> "total_kJ "/1
  Mux/1 -> calc_Power_kW/1
  force_N/1 -> Mux/1
  spd_mps/1 -> Mux/2

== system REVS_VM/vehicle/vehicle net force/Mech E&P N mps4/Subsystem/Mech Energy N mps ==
  force_N : Inport
  spd_mps : Inport  Port=2
  Gain : Gain  Gain=-1
  Integrator : Integrator  ZeroCross=off
  Integrator1 : Integrator  ZeroCross=off
  Integrator2 : Integrator  ZeroCross=off
  Mux : Mux  Inputs=2
  Neg : Fcn  Expr=u(1)*(u(1) <= 0)
  Pos : Fcn  Expr=u(1)*(u(1) >= 0)
  calc_Power_kW : Fcn  Expr=u(1)*u(2)/1000
  "total_kJ " : Outport
  "pos_kJ " : Outport  Port=2
  neg_kJ : Outport  Port=3
  pwr_kW : Outport  Port=4
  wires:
  calc_Power_kW/1 -> Pos/1, Neg/1, pwr_kW/1, Integrator/1
  Gain/1 -> neg_kJ/1
  Integrator1/1 -> "pos_kJ "/1
  Integrator2/1 -> Gain/1
  Neg/1 -> Integrator2/1
  Pos/1 -> Integrator1/1
  Integrator/1 -> "total_kJ "/1
  Mux/1 -> calc_Power_kW/1
  force_N/1 -> Mux/1
  spd_mps/1 -> Mux/2

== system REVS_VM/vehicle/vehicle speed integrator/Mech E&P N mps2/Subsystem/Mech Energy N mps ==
  force_N : Inport
  spd_mps : Inport  Port=2
  Gain : Gain  Gain=-1
  Integrator : Integrator  ZeroCross=off
  Integrator1 : Integrator  ZeroCross=off
  Integrator2 : Integrator  ZeroCross=off
  Mux : Mux  Inputs=2
  Neg : Fcn  Expr=u(1)*(u(1) <= 0)
  Pos : Fcn  Expr=u(1)*(u(1) >= 0)
  calc_Power_kW : Fcn  Expr=u(1)*u(2)/1000
  "total_kJ " : Outport
  "pos_kJ " : Outport  Port=2
  neg_kJ : Outport  Port=3
  pwr_kW : Outport  Port=4
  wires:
  calc_Power_kW/1 -> Pos/1, Neg/1, pwr_kW/1, Integrator/1
  Gain/1 -> neg_kJ/1
  Integrator1/1 -> "pos_kJ "/1
  Integrator2/1 -> Gain/1
  Neg/1 -> Integrator2/1
  Pos/1 -> Integrator1/1
  Integrator/1 -> "total_kJ "/1
  Mux/1 -> calc_Power_kW/1
  force_N/1 -> Mux/1
  spd_mps/1 -> Mux/2

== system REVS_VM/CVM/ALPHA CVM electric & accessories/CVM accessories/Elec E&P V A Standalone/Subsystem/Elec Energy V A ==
  volts_V : Inport
  curr_A : Inport  Port=2
  Gain : Gain  Gain=-1
  Integrator : Integrator  ZeroCross=off
  Integrator1 : Integrator  ZeroCross=off
  Integrator2 : Integrator  ZeroCross=off
  Mux : Mux  Inputs=2
  Neg : Fcn  Expr=u(1)*(u(1) <= 0)
  Pos : Fcn  Expr=u(1)*(u(1) >= 0)
  calc_Power_kW : Fcn  Expr=u(1)*u(2)/1000
  "total_kJ " : Outport
  "pos_kJ " : Outport  Port=2
  neg_kJ : Outport  Port=3
  pwr_kW : Outport  Port=4
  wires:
  curr_A/1 -> Mux/2
  volts_V/1 -> Mux/1
  Mux/1 -> calc_Power_kW/1
  Integrator/1 -> "total_kJ "/1
  Pos/1 -> Integrator1/1
  Neg/1 -> Integrator2/1
  Integrator2/1 -> Gain/1
  Integrator1/1 -> "pos_kJ "/1
  Gain/1 -> neg_kJ/1
  calc_Power_kW/1 -> Integrator/1, pwr_kW/1, Neg/1, Pos/1

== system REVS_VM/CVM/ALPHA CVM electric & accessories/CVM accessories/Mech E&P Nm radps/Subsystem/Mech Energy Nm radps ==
  trq_Nm : Inport
  spd_radps : Inport  Port=2
  Gain : Gain  Gain=-1
  Integrator : Integrator  ZeroCross=off
  Integrator1 : Integrator  ZeroCross=off
  Integrator2 : Integrator  ZeroCross=off
  Mux : Mux  Inputs=2
  Neg : Fcn  Expr=u(1)*(u(1) <= 0)
  Pos : Fcn  Expr=u(1)*(u(1) >= 0)
  calc_Power_kW : Fcn  Expr=u(1)*u(2)/1000
  "total_kJ " : Outport
  "pos_kJ " : Outport  Port=2
  neg_kJ : Outport  Port=3
  pwr_kW : Outport  Port=4
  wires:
  calc_Power_kW/1 -> Pos/1, Neg/1, pwr_kW/1, Integrator/1
  Gain/1 -> neg_kJ/1
  Integrator1/1 -> "pos_kJ "/1
  Integrator2/1 -> Gain/1
  Neg/1 -> Integrator2/1
  Pos/1 -> Integrator1/1
  spd_radps/1 -> Mux/2
  trq_Nm/1 -> Mux/1
  Mux/1 -> calc_Power_kW/1
  Integrator/1 -> "total_kJ "/1

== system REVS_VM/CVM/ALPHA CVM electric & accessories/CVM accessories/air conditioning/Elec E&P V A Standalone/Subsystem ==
  volts_V : Inport
  curr_A : Inport  Port=2
  Enable : EnablePort  ZeroCross=off
  Elec Energy V A : Subsystem  TreatAsAtomicUnit=on
  amps_to_workspace : ToWorkspace  VariableName=audit__elec__accessories__air_conditioner_Amps  SampleTime=-1
  energy_to_workspace : ToWorkspace  VariableName=audit__elec__accessories__air_conditioner_kJ  SampleTime=-1
  neg_energy_to_workspace : ToWorkspace  VariableName=audit__elec__accessories__air_conditioner_neg_kJ  SampleTime=-1
  pos_energy_to_workspace : ToWorkspace  VariableName=audit__elec__accessories__air_conditioner_pos_kJ  SampleTime=-1
  power_to_workspace : ToWorkspace  VariableName=audit__elec__accessories__air_conditioner_kW  SampleTime=-1
  volts_to_workspace : ToWorkspace  VariableName=audit__elec__accessories__air_conditioner_Volts  SampleTime=-1
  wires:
  volts_V/1 -> Elec Energy V A/1(volts_V), volts_to_workspace/1
  curr_A/1 -> Elec Energy V A/2(curr_A), amps_to_workspace/1
  Elec Energy V A/3(neg_kJ) -> neg_energy_to_workspace/1
  Elec Energy V A/2("pos_kJ ") -> pos_energy_to_workspace/1
  Elec Energy V A/4(pwr_kW) -> power_to_workspace/1
  Elec Energy V A/1("total_kJ ") -> energy_to_workspace/1

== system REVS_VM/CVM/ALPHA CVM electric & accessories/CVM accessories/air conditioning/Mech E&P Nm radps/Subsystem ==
  " trq_Nm" : Inport
  spd_radps : Inport  Port=2
  iner_kgm2 : Inport  Port=3
  Enable : EnablePort  ZeroCross=off
  KE_to_workspace : ToWorkspace  VariableName=audit__mech__accessories__air_conditioner_KE_kJ  SampleTime=-1
  Mech Energy Nm radps : Subsystem  TreatAsAtomicUnit=on
  Mult : Product  Inputs=**
  Square : Math  Operator=square
  energy_to_workspace : ToWorkspace  VariableName=audit__mech__accessories__air_conditioner_kJ  SampleTime=-1
  inertia_to_workspace : ToWorkspace  VariableName=audit__mech__accessories__air_conditioner_kgm2  SampleTime=-1
  neg_energy_to_workspace : ToWorkspace  VariableName=audit__mech__accessories__air_conditioner_neg_kJ  SampleTime=-1
  one half : Gain  Gain=0.5/1000
  pos_energy_to_workspace : ToWorkspace  VariableName=audit__mech__accessories__air_conditioner_pos_kJ  SampleTime=-1
  power_to_workspace : ToWorkspace  VariableName=audit__mech__accessories__air_conditioner_kW  SampleTime=-1
  speed_to_workspace : ToWorkspace  VariableName=audit__mech__accessories__air_conditioner_radps  SampleTime=-1
  torque_to_workspace : ToWorkspace  VariableName=audit__mech__accessories__air_conditioner_Nm  SampleTime=-1
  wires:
  Mult/1 -> one half/1
  Square/1 -> Mult/1
  one half/1 -> KE_to_workspace/1
  Mech Energy Nm radps/3(neg_kJ) -> neg_energy_to_workspace/1
  Mech Energy Nm radps/2("pos_kJ ") -> pos_energy_to_workspace/1
  Mech Energy Nm radps/4(pwr_kW) -> power_to_workspace/1
  Mech Energy Nm radps/1("total_kJ ") -> energy_to_workspace/1
  iner_kgm2/1 -> inertia_to_workspace/1, Mult/2
  spd_radps/1 -> Mech Energy Nm radps/2(spd_radps), speed_to_workspace/1, Square/1
  " trq_Nm"/1 -> Mech Energy Nm radps/1(trq_Nm), torque_to_workspace/1

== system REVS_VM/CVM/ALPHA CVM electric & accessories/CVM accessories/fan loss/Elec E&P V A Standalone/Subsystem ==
  volts_V : Inport
  curr_A : Inport  Port=2
  Enable : EnablePort  ZeroCross=off
  Elec Energy V A : Subsystem  TreatAsAtomicUnit=on
  amps_to_workspace : ToWorkspace  VariableName=audit__elec__accessories__fan_Amps  SampleTime=-1
  energy_to_workspace : ToWorkspace  VariableName=audit__elec__accessories__fan_kJ  SampleTime=-1
  neg_energy_to_workspace : ToWorkspace  VariableName=audit__elec__accessories__fan_neg_kJ  SampleTime=-1
  pos_energy_to_workspace : ToWorkspace  VariableName=audit__elec__accessories__fan_pos_kJ  SampleTime=-1
  power_to_workspace : ToWorkspace  VariableName=audit__elec__accessories__fan_kW  SampleTime=-1
  volts_to_workspace : ToWorkspace  VariableName=audit__elec__accessories__fan_Volts  SampleTime=-1
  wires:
  volts_V/1 -> Elec Energy V A/1(volts_V), volts_to_workspace/1
  curr_A/1 -> Elec Energy V A/2(curr_A), amps_to_workspace/1
  Elec Energy V A/3(neg_kJ) -> neg_energy_to_workspace/1
  Elec Energy V A/2("pos_kJ ") -> pos_energy_to_workspace/1
  Elec Energy V A/4(pwr_kW) -> power_to_workspace/1
  Elec Energy V A/1("total_kJ ") -> energy_to_workspace/1

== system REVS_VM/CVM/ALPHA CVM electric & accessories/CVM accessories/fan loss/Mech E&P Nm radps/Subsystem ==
  " trq_Nm" : Inport
  spd_radps : Inport  Port=2
  iner_kgm2 : Inport  Port=3
  Enable : EnablePort  ZeroCross=off
  KE_to_workspace : ToWorkspace  VariableName=audit__mech__accessories__fan_KE_kJ  SampleTime=-1
  Mech Energy Nm radps : Subsystem  TreatAsAtomicUnit=on
  Mult : Product  Inputs=**
  Square : Math  Operator=square
  energy_to_workspace : ToWorkspace  VariableName=audit__mech__accessories__fan_kJ  SampleTime=-1
  inertia_to_workspace : ToWorkspace  VariableName=audit__mech__accessories__fan_kgm2  SampleTime=-1
  neg_energy_to_workspace : ToWorkspace  VariableName=audit__mech__accessories__fan_neg_kJ  SampleTime=-1
  one half : Gain  Gain=0.5/1000
  pos_energy_to_workspace : ToWorkspace  VariableName=audit__mech__accessories__fan_pos_kJ  SampleTime=-1
  power_to_workspace : ToWorkspace  VariableName=audit__mech__accessories__fan_kW  SampleTime=-1
  speed_to_workspace : ToWorkspace  VariableName=audit__mech__accessories__fan_radps  SampleTime=-1
  torque_to_workspace : ToWorkspace  VariableName=audit__mech__accessories__fan_Nm  SampleTime=-1
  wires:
  Mult/1 -> one half/1
  Square/1 -> Mult/1
  one half/1 -> KE_to_workspace/1
  Mech Energy Nm radps/3(neg_kJ) -> neg_energy_to_workspace/1
  Mech Energy Nm radps/2("pos_kJ ") -> pos_energy_to_workspace/1
  Mech Energy Nm radps/4(pwr_kW) -> power_to_workspace/1
  Mech Energy Nm radps/1("total_kJ ") -> energy_to_workspace/1
  iner_kgm2/1 -> inertia_to_workspace/1, Mult/2
  spd_radps/1 -> Mech Energy Nm radps/2(spd_radps), speed_to_workspace/1, Square/1
  " trq_Nm"/1 -> Mech Energy Nm radps/1(trq_Nm), torque_to_workspace/1

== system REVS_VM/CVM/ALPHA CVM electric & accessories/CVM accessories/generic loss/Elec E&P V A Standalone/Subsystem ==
  volts_V : Inport
  curr_A : Inport  Port=2
  Enable : EnablePort  ZeroCross=off
  Elec Energy V A : Subsystem  TreatAsAtomicUnit=on
  amps_to_workspace : ToWorkspace  VariableName=audit__elec__accessories__generic_loss_Amps  SampleTime=-1
  energy_to_workspace : ToWorkspace  VariableName=audit__elec__accessories__generic_loss_kJ  SampleTime=-1
  neg_energy_to_workspace : ToWorkspace  VariableName=audit__elec__accessories__generic_loss_neg_kJ  SampleTime=-1
  pos_energy_to_workspace : ToWorkspace  VariableName=audit__elec__accessories__generic_loss_pos_kJ  SampleTime=-1
  power_to_workspace : ToWorkspace  VariableName=audit__elec__accessories__generic_loss_kW  SampleTime=-1
  volts_to_workspace : ToWorkspace  VariableName=audit__elec__accessories__generic_loss_Volts  SampleTime=-1
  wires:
  volts_V/1 -> Elec Energy V A/1(volts_V), volts_to_workspace/1
  curr_A/1 -> Elec Energy V A/2(curr_A), amps_to_workspace/1
  Elec Energy V A/3(neg_kJ) -> neg_energy_to_workspace/1
  Elec Energy V A/2("pos_kJ ") -> pos_energy_to_workspace/1
  Elec Energy V A/4(pwr_kW) -> power_to_workspace/1
  Elec Energy V A/1("total_kJ ") -> energy_to_workspace/1

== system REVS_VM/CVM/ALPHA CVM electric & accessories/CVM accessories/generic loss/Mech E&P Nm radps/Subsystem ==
  " trq_Nm" : Inport
  spd_radps : Inport  Port=2
  iner_kgm2 : Inport  Port=3
  Enable : EnablePort  ZeroCross=off
  KE_to_workspace : ToWorkspace  VariableName=audit__mech__accessories__generic_loss_KE_kJ  SampleTime=-1
  Mech Energy Nm radps : Subsystem  TreatAsAtomicUnit=on
  Mult : Product  Inputs=**
  Square : Math  Operator=square
  energy_to_workspace : ToWorkspace  VariableName=audit__mech__accessories__generic_loss_kJ  SampleTime=-1
  inertia_to_workspace : ToWorkspace  VariableName=audit__mech__accessories__generic_loss_kgm2  SampleTime=-1
  neg_energy_to_workspace : ToWorkspace  VariableName=audit__mech__accessories__generic_loss_neg_kJ  SampleTime=-1
  one half : Gain  Gain=0.5/1000
  pos_energy_to_workspace : ToWorkspace  VariableName=audit__mech__accessories__generic_loss_pos_kJ  SampleTime=-1
  power_to_workspace : ToWorkspace  VariableName=audit__mech__accessories__generic_loss_kW  SampleTime=-1
  speed_to_workspace : ToWorkspace  VariableName=audit__mech__accessories__generic_loss_radps  SampleTime=-1
  torque_to_workspace : ToWorkspace  VariableName=audit__mech__accessories__generic_loss_Nm  SampleTime=-1
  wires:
  Mult/1 -> one half/1
  Square/1 -> Mult/1
  one half/1 -> KE_to_workspace/1
  Mech Energy Nm radps/3(neg_kJ) -> neg_energy_to_workspace/1
  Mech Energy Nm radps/2("pos_kJ ") -> pos_energy_to_workspace/1
  Mech Energy Nm radps/4(pwr_kW) -> power_to_workspace/1
  Mech Energy Nm radps/1("total_kJ ") -> energy_to_workspace/1
  iner_kgm2/1 -> inertia_to_workspace/1, Mult/2
  spd_radps/1 -> Mech Energy Nm radps/2(spd_radps), speed_to_workspace/1, Square/1
  " trq_Nm"/1 -> Mech Energy Nm radps/1(trq_Nm), torque_to_workspace/1

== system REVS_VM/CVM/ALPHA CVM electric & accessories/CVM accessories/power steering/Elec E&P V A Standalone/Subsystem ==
  volts_V : Inport
  curr_A : Inport  Port=2
  Enable : EnablePort  ZeroCross=off
  Elec Energy V A : Subsystem  TreatAsAtomicUnit=on
  amps_to_workspace : ToWorkspace  VariableName=audit__elec__accessories__power_steering_Amps  SampleTime=-1
  energy_to_workspace : ToWorkspace  VariableName=audit__elec__accessories__power_steering_kJ  SampleTime=-1
  neg_energy_to_workspace : ToWorkspace  VariableName=audit__elec__accessories__power_steering_neg_kJ  SampleTime=-1
  pos_energy_to_workspace : ToWorkspace  VariableName=audit__elec__accessories__power_steering_pos_kJ  SampleTime=-1
  power_to_workspace : ToWorkspace  VariableName=audit__elec__accessories__power_steering_kW  SampleTime=-1
  volts_to_workspace : ToWorkspace  VariableName=audit__elec__accessories__power_steering_Volts  SampleTime=-1
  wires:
  volts_V/1 -> Elec Energy V A/1(volts_V), volts_to_workspace/1
  curr_A/1 -> Elec Energy V A/2(curr_A), amps_to_workspace/1
  Elec Energy V A/3(neg_kJ) -> neg_energy_to_workspace/1
  Elec Energy V A/2("pos_kJ ") -> pos_energy_to_workspace/1
  Elec Energy V A/4(pwr_kW) -> power_to_workspace/1
  Elec Energy V A/1("total_kJ ") -> energy_to_workspace/1

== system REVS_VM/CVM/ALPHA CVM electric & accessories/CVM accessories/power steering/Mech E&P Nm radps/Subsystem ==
  " trq_Nm" : Inport
  spd_radps : Inport  Port=2
  iner_kgm2 : Inport  Port=3
  Enable : EnablePort  ZeroCross=off
  KE_to_workspace : ToWorkspace  VariableName=audit__mech__accessories__power_steering_KE_kJ  SampleTime=-1
  Mech Energy Nm radps : Subsystem  TreatAsAtomicUnit=on
  Mult : Product  Inputs=**
  Square : Math  Operator=square
  energy_to_workspace : ToWorkspace  VariableName=audit__mech__accessories__power_steering_kJ  SampleTime=-1
  inertia_to_workspace : ToWorkspace  VariableName=audit__mech__accessories__power_steering_kgm2  SampleTime=-1
  neg_energy_to_workspace : ToWorkspace  VariableName=audit__mech__accessories__power_steering_neg_kJ  SampleTime=-1
  one half : Gain  Gain=0.5/1000
  pos_energy_to_workspace : ToWorkspace  VariableName=audit__mech__accessories__power_steering_pos_kJ  SampleTime=-1
  power_to_workspace : ToWorkspace  VariableName=audit__mech__accessories__power_steering_kW  SampleTime=-1
  speed_to_workspace : ToWorkspace  VariableName=audit__mech__accessories__power_steering_radps  SampleTime=-1
  torque_to_workspace : ToWorkspace  VariableName=audit__mech__accessories__power_steering_Nm  SampleTime=-1
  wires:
  Mult/1 -> one half/1
  Square/1 -> Mult/1
  one half/1 -> KE_to_workspace/1
  Mech Energy Nm radps/3(neg_kJ) -> neg_energy_to_workspace/1
  Mech Energy Nm radps/2("pos_kJ ") -> pos_energy_to_workspace/1
  Mech Energy Nm radps/4(pwr_kW) -> power_to_workspace/1
  Mech Energy Nm radps/1("total_kJ ") -> energy_to_workspace/1
  iner_kgm2/1 -> inertia_to_workspace/1, Mult/2
  spd_radps/1 -> Mech Energy Nm radps/2(spd_radps), speed_to_workspace/1, Square/1
  " trq_Nm"/1 -> Mech Energy Nm radps/1(trq_Nm), torque_to_workspace/1

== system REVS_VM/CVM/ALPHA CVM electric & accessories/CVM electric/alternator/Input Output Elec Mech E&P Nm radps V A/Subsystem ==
  volts_in_V : Inport
  curr_in_A : Inport  Port=2
  trq_out_Nm : Inport  Port=3
  spd_out_radps : Inport  Port=4
  iner_out_kgm2 : Inport  Port=5
  Enable : EnablePort
  Elec E&P V A : Subsystem
  Loss_KJ_to_workspace : ToWorkspace  VariableName=audit__mech__alternator__loss_kJ  SampleTime=-1
  Mech E&P Nm radps : Subsystem
  Pos : Saturate  UpperLimit=Inf  LowerLimit=0  ZeroCross=off
  Pos2 : Saturate  UpperLimit=Inf  LowerLimit=0  ZeroCross=off
  Sum : Sum  Inputs=+-|
  Sum1 : Sum  Inputs=|-+
  Sum2 : Sum
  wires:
  Pos2/1 -> Sum2/1
  Pos/1 -> Sum2/2
  trq_out_Nm/1 -> Mech E&P Nm radps/1(" trq_Nm")
  spd_out_radps/1 -> Mech E&P Nm radps/2(spd_radps)
  volts_in_V/1 -> Elec E&P V A/1(volts_V)
  curr_in_A/1 -> Elec E&P V A/2(curr_A)
  iner_out_kgm2/1 -> Mech E&P Nm radps/3(iner_kgm2)
  Mech E&P Nm radps/1(pos_kJ) -> Sum/2
  Elec E&P V A/2(neg_kJ) -> Sum1/1
  Mech E&P Nm radps/2(neg_kJ) -> Sum1/2
  Sum/1 -> Pos/1
  Sum1/1 -> Pos2/1
  Sum2/1 -> Loss_KJ_to_workspace/1
  Elec E&P V A/1(pos_kJ) -> Sum/1
